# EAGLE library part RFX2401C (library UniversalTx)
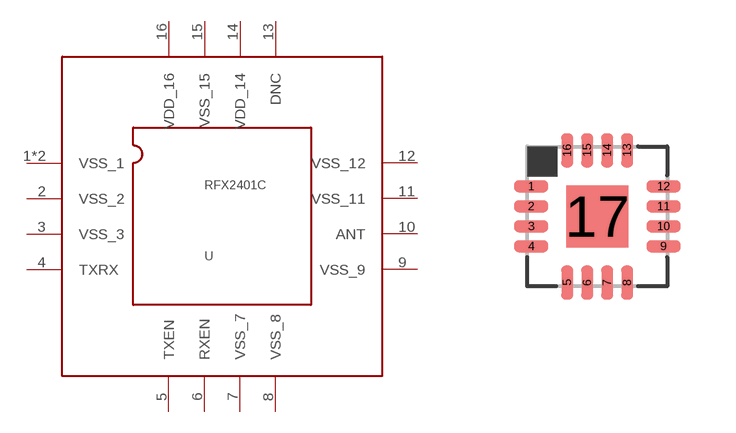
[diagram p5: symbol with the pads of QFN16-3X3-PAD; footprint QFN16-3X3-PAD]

Designator prefix -

## RFX2401C  [QFN16-3X3-PAD]
1  VSS_1
2  VSS_2
3  VSS_3
4  TXRX
5  TXEN
6  RXEN
7  VSS_7
8  VSS_8
9  VSS_9
10  ANT
11  VSS_11
12  VSS_12
13  DNC
14  VDD_14
15  VSS_15
16  VDD_16
17  VSS_1

## Footprint QFN16-3X3-PAD (pad centres in mm)
RTE (S-PQFP-N16) 3x3 mm Source: www.ti.com .. tpa6132a2 direct path stereo $.65.pdf
smd 0.85 x 0.3: 1 -1.655,0.75; 2 -1.655,0.25; 3 -1.655,-0.25; 4 -1.655,-0.75; 9 1.655,-0.75; 10 1.655,-0.25; 11 1.655,0.25; 12 1.655,0.75
smd 0.3 x 0.85: 5 -0.75,-1.655; 6 -0.25,-1.655; 7 0.25,-1.655; 8 0.75,-1.655; 13 0.75,1.655; 14 0.25,1.655; 15 -0.25,1.655; 16 -0.75,1.655
smd 1.55 x 1.55: 17 0,0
